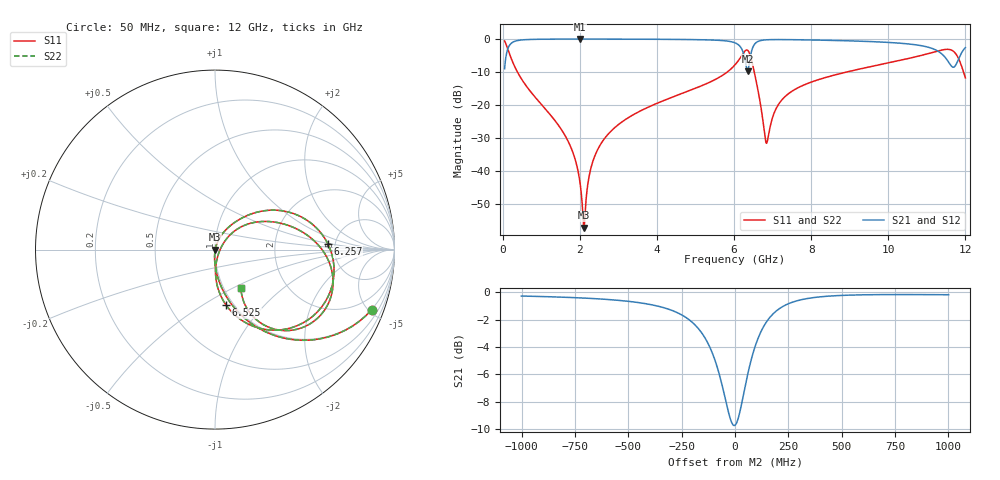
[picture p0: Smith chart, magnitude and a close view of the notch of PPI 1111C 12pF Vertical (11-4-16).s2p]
# GHz S MA R 50
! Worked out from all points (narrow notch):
!   1601 points, 50 MHz to 12 GHz, reference 50 ohm
!   highest |S21| = -0.01 dB at 2.007 GHz (marker M1); lowest = -9.7 dB at 6.354 GHz (marker M2)
!   notch at M2: 9.5 dB deep, 168 MHz wide at half that depth
!   lowest |S11| = -57.2 dB at 2.104 GHz (marker M3), VSWR 1.00, Z = 50.1 - j0.0468 ohm
!   |S11| at or under -10 dB: 382.9 MHz to 5.823 GHz (5.44 GHz wide, 175 % of centre); 6.525 GHz to 8.917 GHz (2.391 GHz wide, 31 % of centre); 11.95172 GHz to end of sweep
!   |S22| runs from -57.2 to -0.6 dB; largest |S21 - S12| = 0
!   S11 on the Smith chart (normalised r, x): 50 MHz: 0.98, -5.21; 6.257 GHz: 4.35, +0.46; 6.525 GHz: 0.92, -0.63; 12 GHz: 1.20, -0.55
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0.05  0.9349 -21.0  0.3548 69.0  0.3548 69.0  0.9349 -21.0
0.2217813  0.5068 -60.6  0.8616 29.4  0.8616 29.4  0.5068 -60.6
0.4234375  0.2867 -75.2  0.9574 14.6  0.9574 14.6  0.2867 -75.2
1.633375  0.03329 -93.8  0.9981 -5.9  0.9981 -5.9  0.03329 -93.8
1.872375  0.01554 -93.3  0.9985 -8.1  0.9985 -8.1  0.01554 -93.3
2.006813  0.006578 -87.5  0.9985 -9.2  0.9985 -9.2  0.006578 -87.5
2.044156  0.004244 -81.0  0.9985 -9.5  0.9985 -9.5  0.004244 -81.0
2.103906  0.001388 -19.7  0.9985 -10.0  0.9985 -10.0  0.001388 -19.7
2.305563  0.01209 71.5  0.9983 -11.7  0.9983 -11.7  0.01209 71.5
2.589375  0.02823 72.9  0.9979 -14.0  0.9979 -14.0  0.02823 72.9
4.038312  0.1084 63.5  0.9916 -25.4  0.9916 -25.4  0.1084 63.5
6.025  0.4067 32.6  0.8764 -52.1  0.8764 -52.1  0.4067 32.6
6.256531  0.6297 2.9  0.5738 -64.9  0.5738 -64.9  0.6297 2.9
6.353625  0.6747 -28.3  0.3255 -32.4  0.3255 -32.4  0.6747 -28.3
6.525406  0.3156 -78.7  0.824 -13.8  0.824 -13.8  0.3156 -78.7
6.846563  0.02643 -16.7  0.9741 -32.2  0.9741 -32.2  0.02643 -16.7
7.22  0.1158 44.3  0.9815 -40.0  0.9815 -40.0  0.1158 44.3
8.019156  0.2245 38.5  0.9675 -49.8  0.9675 -49.8  0.2245 38.5
10.01331  0.4371 17.5  0.8882 -71.1  0.8882 -71.1  0.4371 17.5
11.44731  0.692 -18.9  0.5508 -92.4  0.5508 -92.4  0.692 -18.9
11.74606  0.6022 -48.5  0.3998 -57.1  0.3998 -57.1  0.6022 -48.5
12  0.2587 -56.1  0.7412 -51.8  0.7412 -51.8  0.2587 -56.1
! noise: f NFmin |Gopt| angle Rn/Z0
0.05  0.0003887  0.8752  1.627  0.0006724
1.372  0.00383  0.6794  6.82  0.002302
2.701  0.006425  0.6363  12.68  0.003289
4.031  0.009329  0.632  18.43  0.004647
5.36  0.01695  0.721  24.48  0.01151
6.682  0.05505  0.8849  31.12  0.09637
8.012  0.02191  0.696  35.95  0.01277
9.341  0.02518  0.7002  40.95  0.01449
10.67  0.04922  0.818  47.01  0.0477
12  0.1806  0.942  52.92  0.5586
